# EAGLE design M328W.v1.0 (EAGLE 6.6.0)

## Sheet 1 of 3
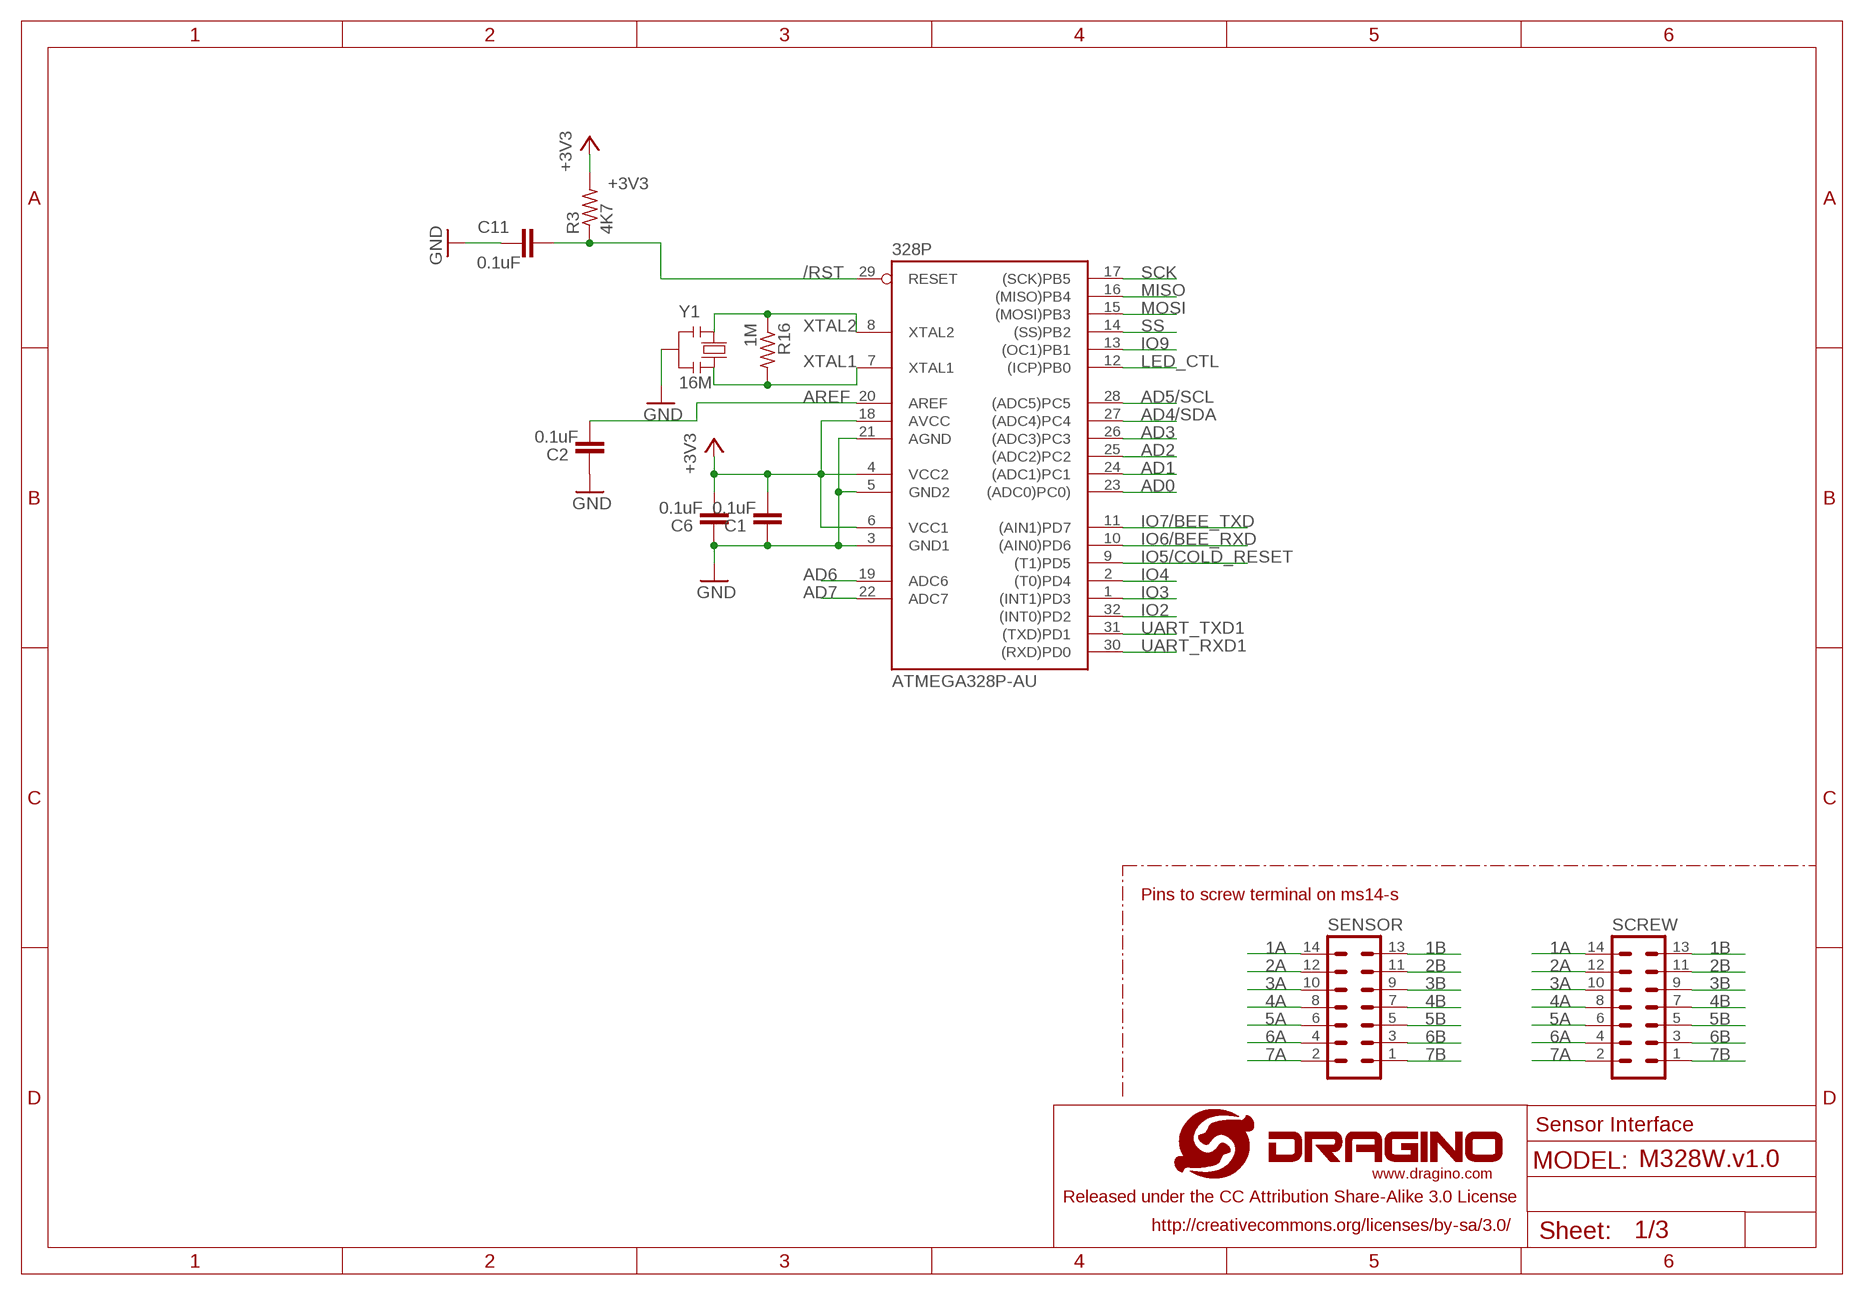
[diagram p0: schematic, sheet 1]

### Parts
328P  ATMEGA328P-AU  [TQFP32-08]
C1  0.1uF  C-EUC0402  [C0402]
C2  0.1uF  C-EUC0402  [C0402]
C6  0.1uF  C-EUC0402  [C0402]
C11  0.1uF  C-EUC0402  [C0402]
R3  4K7  R-US_R0402  [R0402]
R16  1M  R-US_R0402  [R0402]
SCREW  MA07-2  [MA07-2]
SENSOR  MA07-2  [MA07-2]
Y1  16M  RESONATORMU  [RESONATOR]

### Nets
1A: SCREW.14 SENSOR.14
1B: SCREW.13 SENSOR.13
2A: SCREW.12 SENSOR.12
2B: SCREW.11 SENSOR.11
3A: SCREW.10 SENSOR.10
3B: SCREW.9 SENSOR.9
4A: SCREW.8 SENSOR.8
4B: SCREW.7 SENSOR.7
5A: SCREW.6 SENSOR.6
5B: SCREW.5 SENSOR.5
6A: SCREW.4 SENSOR.4
6B: SCREW.3 SENSOR.3
7A: SCREW.2 SENSOR.2
7B: SCREW.1 SENSOR.1
+3V3: 328P.4(VCC2) 328P.6(VCC1) 328P.18(AVCC) C1.2 C6.2 R3.2 ; also sheet 2,3
/RST: 328P.29(RESET) C11.1 R3.1 ; also sheet 2
AD0: 328P.23((ADC0)PC0)) ; also sheet 2
AD1: 328P.24((ADC1)PC1) ; also sheet 2
AD2: 328P.25((ADC2)PC2) ; also sheet 2
AD3: 328P.26((ADC3)PC3) ; also sheet 2
AD4/SDA: 328P.27((ADC4)PC4) ; also sheet 2
AD5/SCL: 328P.28((ADC5)PC5) ; also sheet 2
AD6: 328P.19(ADC6)
AD7: 328P.22(ADC7)
AREF: 328P.20(AREF) C2.2 ; also sheet 2
GND [gnd]: 328P.3(GND1) 328P.5(GND2) 328P.21(AGND) C1.1 C2.1 C6.1 C11.2 Y1.2 ; also sheet 2,3
IO2: 328P.32((INT0)PD2) ; also sheet 2,3
IO3: 328P.1((INT1)PD3) ; also sheet 2
IO4: 328P.2((T0)PD4) ; also sheet 2
IO5/COLD_RESET: 328P.9((T1)PD5) ; also sheet 2
IO6/BEE_RXD: 328P.10((AIN0)PD6) ; also sheet 2,3
IO7/BEE_TXD: 328P.11((AIN1)PD7) ; also sheet 2,3
IO9: 328P.13((OC1)PB1) ; also sheet 2
LED_CTL: 328P.12((ICP)PB0) ; also sheet 2
MISO: 328P.16((MISO)PB4) ; also sheet 2,3
MOSI: 328P.15((MOSI)PB3) ; also sheet 2,3
SCK: 328P.17((SCK)PB5) ; also sheet 2,3
SS: 328P.14((SS)PB2) ; also sheet 2,3
UART_RXD1: 328P.30((RXD)PD0) ; also sheet 2
UART_TXD1: 328P.31((TXD)PD1) ; also sheet 2
XTAL1: 328P.7(XTAL1) R16.2 Y1.3
XTAL2: 328P.8(XTAL2) R16.1 Y1.1

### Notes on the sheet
- Pins to screw terminal on ms14-s
- Sensor Interface

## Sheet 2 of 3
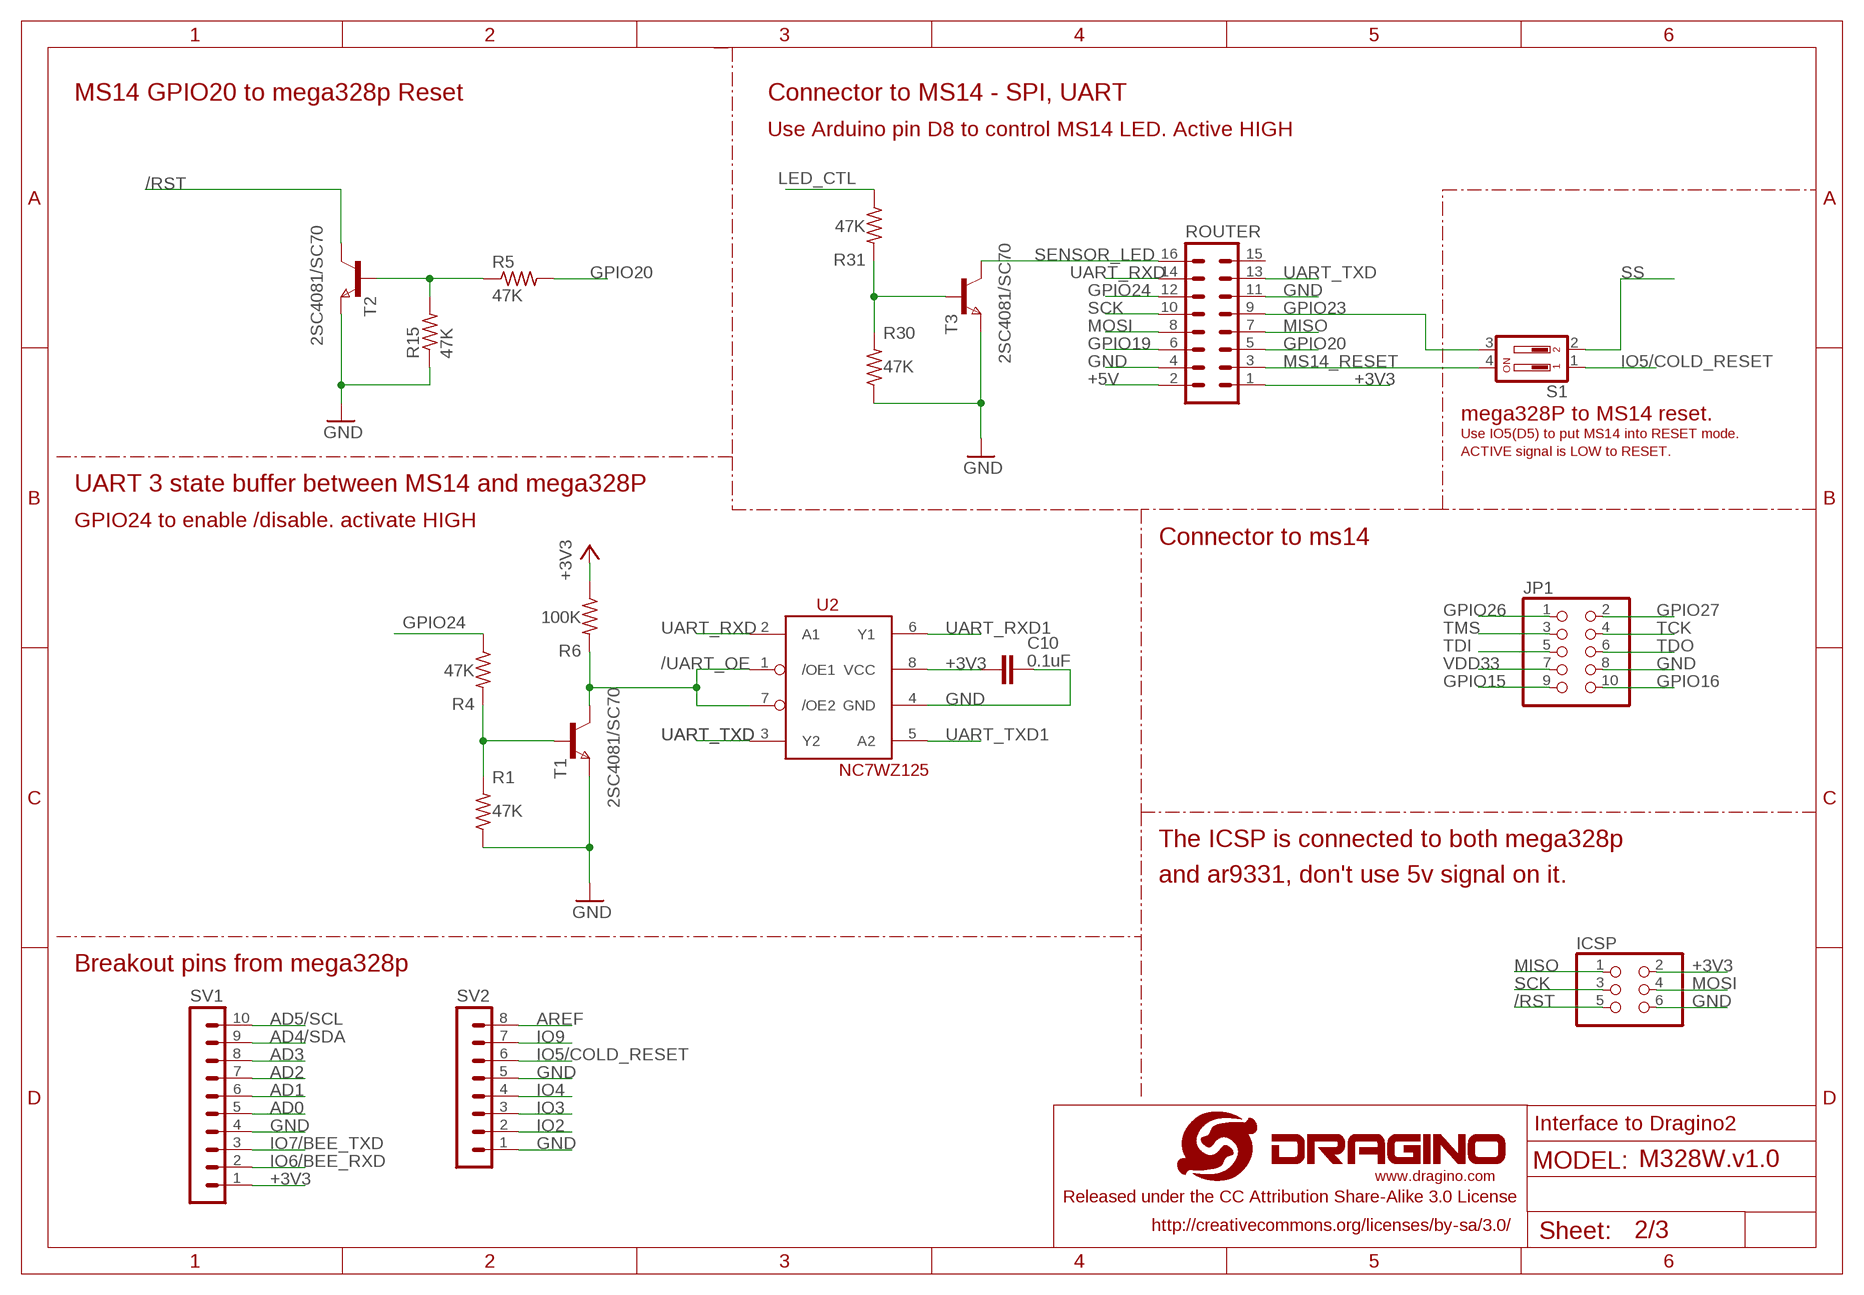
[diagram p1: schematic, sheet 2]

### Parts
C10  0.1uF  C-EUC0402  [C0402]
ICSP  PINHD-2X3  [2X03]
JP1  PINHD-2X5_2.00  [2X05M]
R1  47K  R-US_R0402  [R0402]
R4  47K  R-US_R0402  [R0402]
R5  47K  R-US_R0402  [R0402]
R6  100K  R-US_R0402  [R0402]
R15  47K  R-US_R0402  [R0402]
R30  47K  R-US_R0402  [R0402]
R31  47K  R-US_R0402  [R0402]
ROUTER  MA08-2  [MA08-2]
S1  DIP02YL  [DIP02YL]
SV1  MA10-1  [MA10-1]
SV2  MA08-1  [MA08-1]
T1  2SC4081/SC70  NPNSOT323  [SOT323]
T2  2SC4081/SC70  NPNSOT323  [SOT323]
T3  2SC4081/SC70  NPNSOT323  [SOT323]
U2  NC7WZ125  [US8]
U$5  LOGO-NEW  [LOGO-SILK-NEW]

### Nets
+3V3: C10.2 ICSP.2 R6.1 ROUTER.1 SV1.1 U2.8(VCC) ; also sheet 1,3
+5V: ROUTER.2
/RST: ICSP.5 T2.1(C) ; also sheet 1
/UART_OE: R6.2 T1.1(C) U2.1(/OE1) U2.7(/OE2)
AD0: SV1.5 ; also sheet 1
AD1: SV1.6 ; also sheet 1
AD2: SV1.7 ; also sheet 1
AD3: SV1.8 ; also sheet 1
AD4/SDA: SV1.9 ; also sheet 1
AD5/SCL: SV1.10 ; also sheet 1
AREF: SV2.8 ; also sheet 1
GND [gnd]: C10.1 ICSP.6 JP1.8 R1.1 R15.1 R30.1 ROUTER.4 ROUTER.11 SV1.4 SV2.1 SV2.5 T1.3(E) T2.3(E) T3.3(E) U2.4(GND) ; also sheet 1,3
GPIO15: JP1.9
GPIO16: JP1.10
GPIO19: ROUTER.6
GPIO20: R5.2 ROUTER.5
GPIO23: ROUTER.9 S1.3
GPIO24: R4.1 ROUTER.12
GPIO26: JP1.1 ; also sheet 3
GPIO27: JP1.2 ; also sheet 3
IO2: SV2.2 ; also sheet 1,3
IO3: SV2.3 ; also sheet 1
IO4: SV2.4 ; also sheet 1
IO5/COLD_RESET: S1.1 SV2.6 ; also sheet 1
IO6/BEE_RXD: SV1.2 ; also sheet 1,3
IO7/BEE_TXD: SV1.3 ; also sheet 1,3
IO9: SV2.7 ; also sheet 1
LED_CTL: R31.1 ; also sheet 1
MISO: ICSP.1 ROUTER.7 ; also sheet 1,3
MOSI: ICSP.4 ROUTER.8 ; also sheet 1,3
MS14_RESET: ROUTER.3 S1.4
N$4: R1.2 R4.2 T1.2(B)
N$8: R5.1 R15.2 T2.2(B)
N$9: R30.2 R31.2 T3.2(B)
SCK: ICSP.3 ROUTER.10 ; also sheet 1,3
SENSOR_LED: ROUTER.16 T3.1(C)
SS: S1.2 ; also sheet 1,3
TCK: JP1.4
TDI: JP1.5
TDO: JP1.6
TMS: JP1.3
UART_RXD: ROUTER.14 U2.2(A1) ; also sheet 3
UART_RXD1: U2.6(Y1) ; also sheet 1
UART_TXD: ROUTER.13 U2.3(Y2) ; also sheet 3
UART_TXD1: U2.5(A2) ; also sheet 1
VDD33: JP1.7
Unconnected: ROUTER.15

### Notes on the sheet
- MS14 GPIO20 to mega328p Reset | Connector to MS14 - SPI, UART
- Use Arduino pin D8 to control MS14 LED. Active HIGH
- mega328P to MS14 reset.
- Use IO5(D5) to put MS14 into RESET mode.
- ACTIVE signal is LOW to RESET.
- UART 3 state buffer between MS14 and mega328P
- GPIO24 to enable /disable. activate HIGH
- Connector to ms14
- The ICSP is connected to both mega328p
- and ar9331, don't use 5v signal on it.
- Breakout pins from mega328p
- Interface to Dragino2

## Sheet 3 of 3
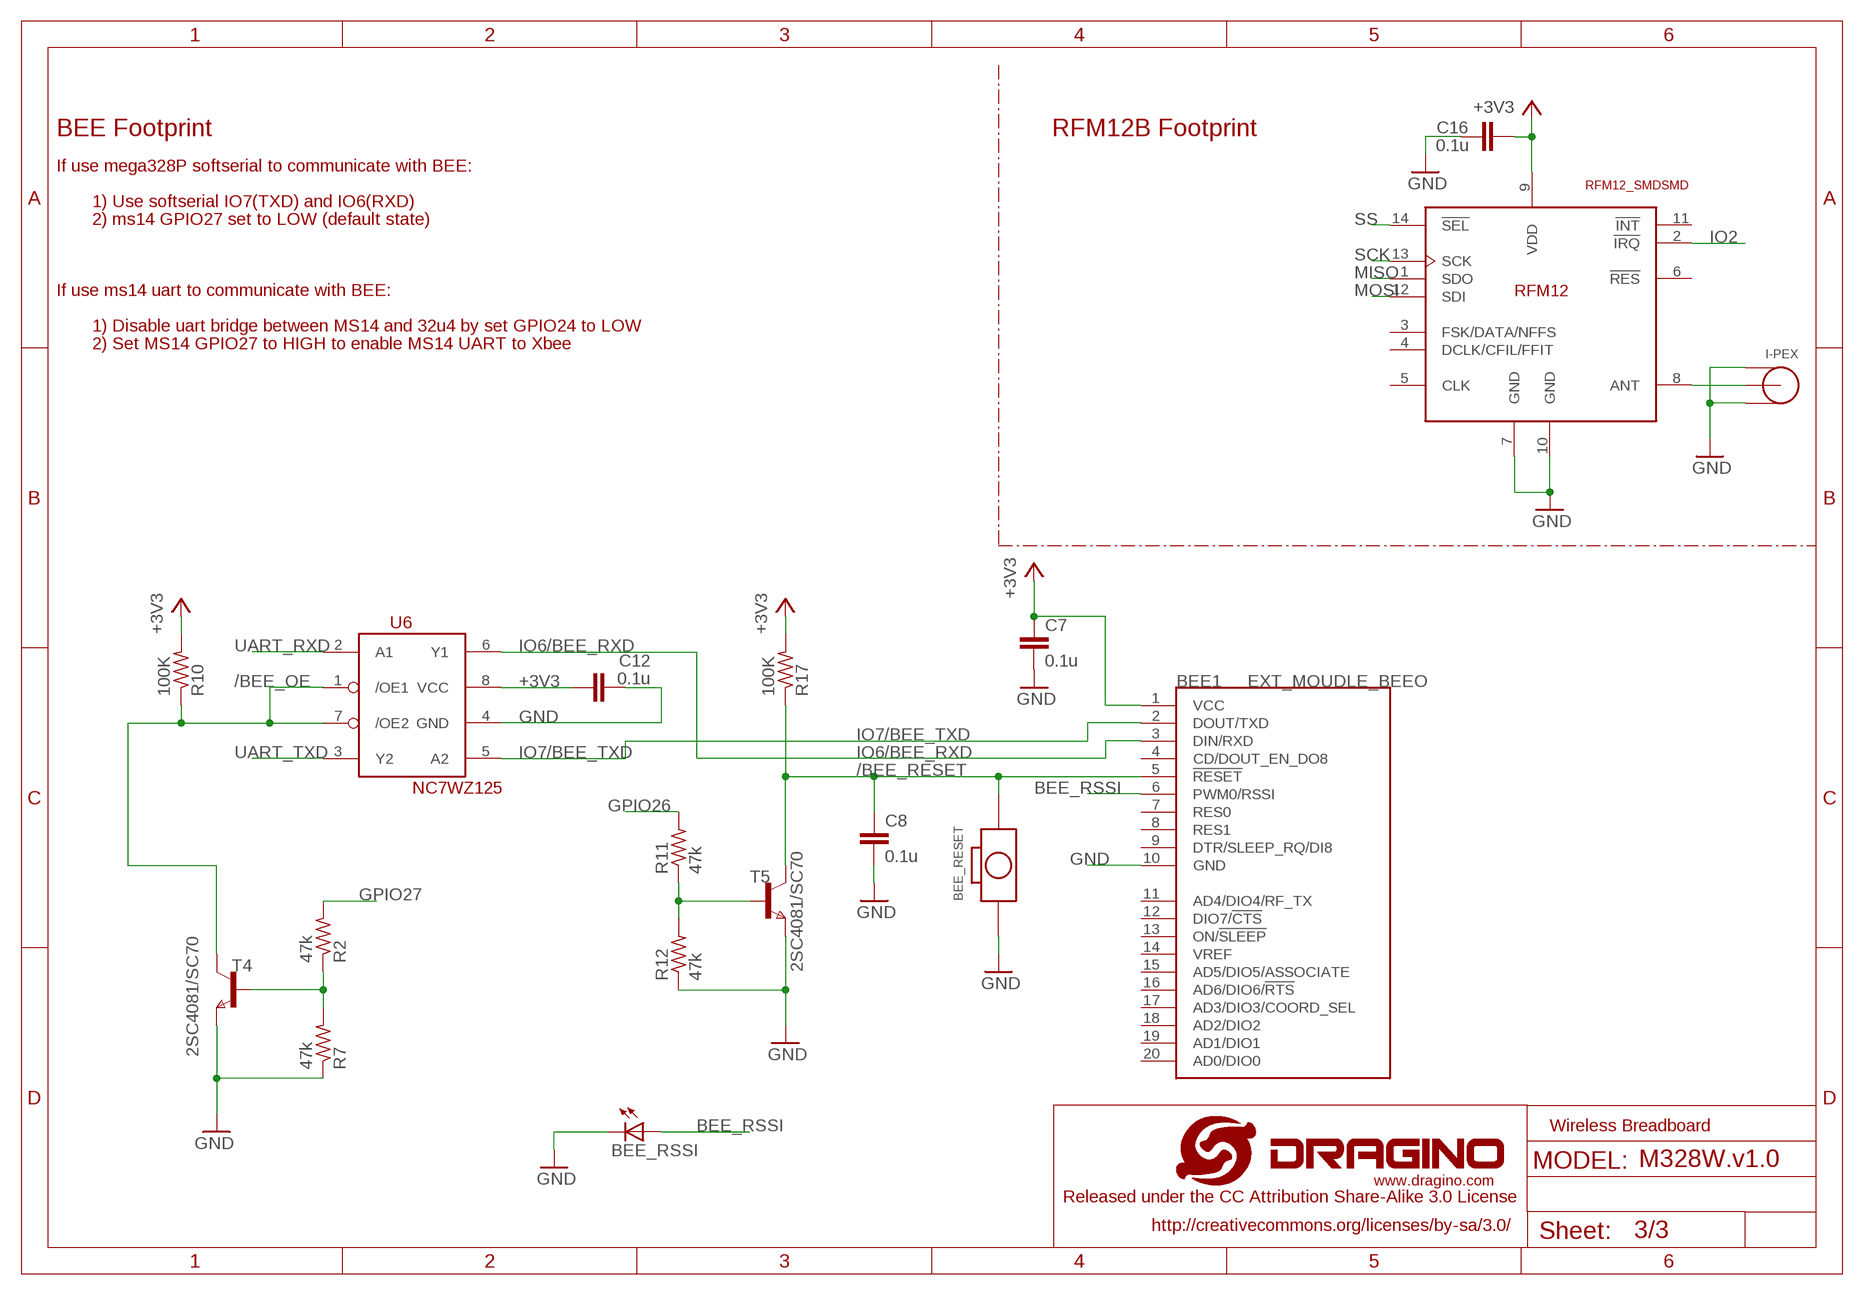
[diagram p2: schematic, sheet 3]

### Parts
BEE1  EXT_MOUDLE_BEEO  [EXT_MOUDLE_BEE]
BEE_RESET  CPT_SMD_BOTTON_1_SMD  [CPT_SMD_BOTTON_1]
BEE_RSSI  LEDCHIP-LED0805  [CHIP-LED0805]
C7  0.1u  C-EUC0402  [C0402]
C8  0.1u  C-EUC0402  [C0402]
C12  0.1u  C-EUC0402  [C0402]
C16  0.1u  C-EUC0402  [C0402]
I-PEX  I-PEX  [I-PEX]
R2  47k  R-US_R0402  [R0402]
R7  47k  R-US_R0402  [R0402]
R10  100K  R-US_R0402  [R0402]
R11  47k  R-US_R0402  [R0402]
R12  47k  R-US_R0402  [R0402]
R17  100K  R-US_R0402  [R0402]
T4  2SC4081/SC70  NPNSOT323  [SOT323]
T5  2SC4081/SC70  NPNSOT323  [SOT323]
U6  NC7WZ125  [US8]
U$3  RFM12_SMDSMD  [RFM12]

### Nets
+3V3: BEE1.1(VCC) C7.1 C12.1 C16.2 R10.2 R17.2 U6.8(VCC) U$3.9(VDD) ; also sheet 1,2
/BEE_OE: R10.1 T4.1(C) U6.1(/OE1) U6.7(/OE2)
/BEE_RESET: BEE1.5(!RESET) BEE_RESET.P$2 C8.1 R17.1 T5.1(C)
BEE_RSSI: BEE1.6(PWM0/RSSI) BEE_RSSI.A
GND [gnd]: BEE1.10(GND) BEE_RESET.1 BEE_RSSI.C C7.2 C8.2 C12.2 C16.1 I-PEX.GND I-PEX.GND1 R7.1 R12.1 T4.3(E) T5.3(E) U6.4(GND) U$3.7(GND) U$3.10(GND) ; also sheet 1,2
GPIO26: R11.2 ; also sheet 2
GPIO27: R2.2 ; also sheet 2
IO2: U$3.2(!IRQ) ; also sheet 1,2
IO6/BEE_RXD: BEE1.3(DIN/RXD) U6.6(Y1) ; also sheet 1,2
IO7/BEE_TXD: BEE1.2(DOUT/TXD) U6.5(A2) ; also sheet 1,2
MISO: U$3.1(SDO) ; also sheet 1,2
MOSI: U$3.12(SDI) ; also sheet 1,2
N$11: R2.1 R7.2 T4.2(B)
N$12: R11.1 R12.2 T5.2(B)
N$16: I-PEX.SIG U$3.8(ANT)
SCK: U$3.13(SCK) ; also sheet 1,2
SS: U$3.14(!SEL) ; also sheet 1,2
UART_RXD: U6.2(A1) ; also sheet 2
UART_TXD: U6.3(Y2) ; also sheet 2
Unconnected: BEE1.4(CD/DOUT_EN_DO8) BEE1.7(RES0) BEE1.8(RES1) BEE1.9(DTR/SLEEP_RQ/DI8) BEE1.11(AD4/DIO4/RF_TX) BEE1.12(DIO7/!CTS) BEE1.13(ON/!SLEEP) BEE1.14(VREF) BEE1.15(AD5/DIO5/ASSOCIATE) BEE1.16(AD6/DIO6/!RTS) BEE1.17(AD3/DIO3/COORD_SEL) BEE1.18(AD2/DIO2) BEE1.19(AD1/DIO1) BEE1.20(AD0/DIO0) U$3.3(FSK/DATA/NFFS) U$3.4(DCLK/CFIL/FFIT) U$3.5(CLK) U$3.6(!RES) U$3.11(!INT)

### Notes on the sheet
- BEE Footprint | RFM12B Footprint
- If use mega328P softserial to communicate with BEE:
- 1) Use softserial IO7(TXD) and IO6(RXD)
- 2) ms14 GPIO27 set to LOW (default state)
- If use ms14 uart to communicate with BEE:
- 1) Disable uart bridge between MS14 and 32u4 by set GPIO24 to LOW
- 2) Set MS14 GPIO27 to HIGH to enable MS14 UART to Xbee
- Wireless Breadboard

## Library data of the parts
328P = dragino:ATMEGA328P-: MICROCONTROLLER 4 Kbytes FLASH 128 bytes SRAM 256 bytes EEPROM UART 6-channel 10 bit ADC
BEE1 = Bees_Shield:EXT_MOUDLE_BEE
BEE_RESET = Bees_Shield:CPT_SMD_BOTTON_1
BEE_RSSI = dragino:LED: LED
C1 C2 C6-C8 C10-C12 C16 = dragino:C-EU: CAPACITOR, European symbol
I-PEX = dragino:I-PEX: I-PEX connector
ICSP = dragino:PINHD-2X3: PIN HEADER
JP1 = dragino:PINHD-2X5: PIN HEADER
R1-R7 R10-R12 R15-R17 R30 R31 = dragino:R-US_: RESISTOR, American symbol
ROUTER = dragino:MA08-2: PIN HEADER; OC_FARNELL: unknown; OC_NEWARK: unknown
S1 = switch-dil:DIP02YL: DIL/CODE SWITCH; OC_FARNELL: unknown; OC_NEWARK: unknown
SCREW SENSOR = dragino:MA07-2: PIN HEADER; OC_FARNELL: unknown; OC_NEWARK: unknown
SV1 = con-lstb:MA10-1: PIN HEADER; OC_FARNELL: unknown; OC_NEWARK: unknown
SV2 = con-lstb:MA08-1: PIN HEADER; OC_FARNELL: unknown; OC_NEWARK: unknown
T1-T5 = zetex:NPNSOT323: NPN TRANSISTOR; MPN: DSS4160U-7; OC_FARNELL: 1710696; OC_NEWARK: 25R4558
U2 U6 = dragino:NC7WZ125: 3 state buffer: http://www.fairchildsemi.com/ds/NC/NC7WZ125.pdf
U$3 = dragino:RFM12_SMD: RFM12 is a low costing ISM band transceiver module implemented with unique PLL. It works signal ranges from 315/433/868/915MHZ bands, comply with FCC, ETSI regulation. The SPI interface is used to communicate with microcontroller for parameter setting.
U$5 = dragino:LOGO-NEW
Y1 = SmartPrj:RESONATOR

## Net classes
0 default: width 0.203 mm, clearance 0.254 mm
1 power: width 0.61 mm, drill 0.61 mm, clearance 0.254 mm
2 gnd: width 0.305 mm, drill 0.33 mm, clearance 0.254 mm
3 usbvcc: width 0.508 mm, drill 0.61 mm, clearance 0.254 mm
4 aref: width 0.406 mm, drill 0.61 mm, clearance 0.254 mm
5 usbtrace: width 0.254 mm, clearance 0.152 mm

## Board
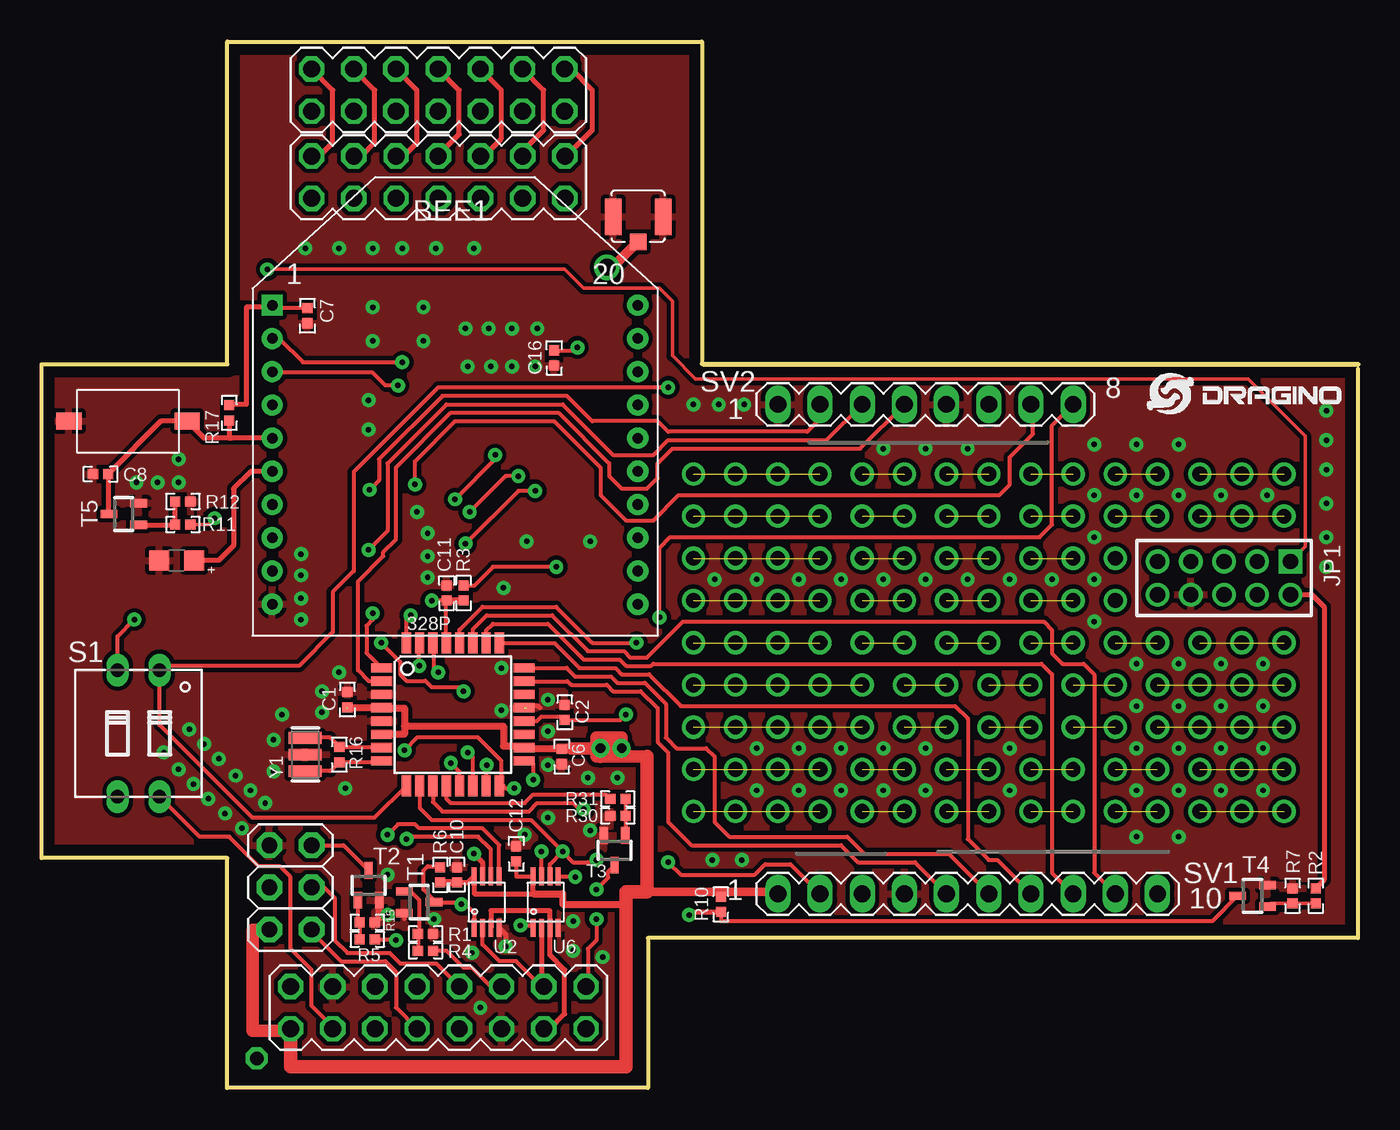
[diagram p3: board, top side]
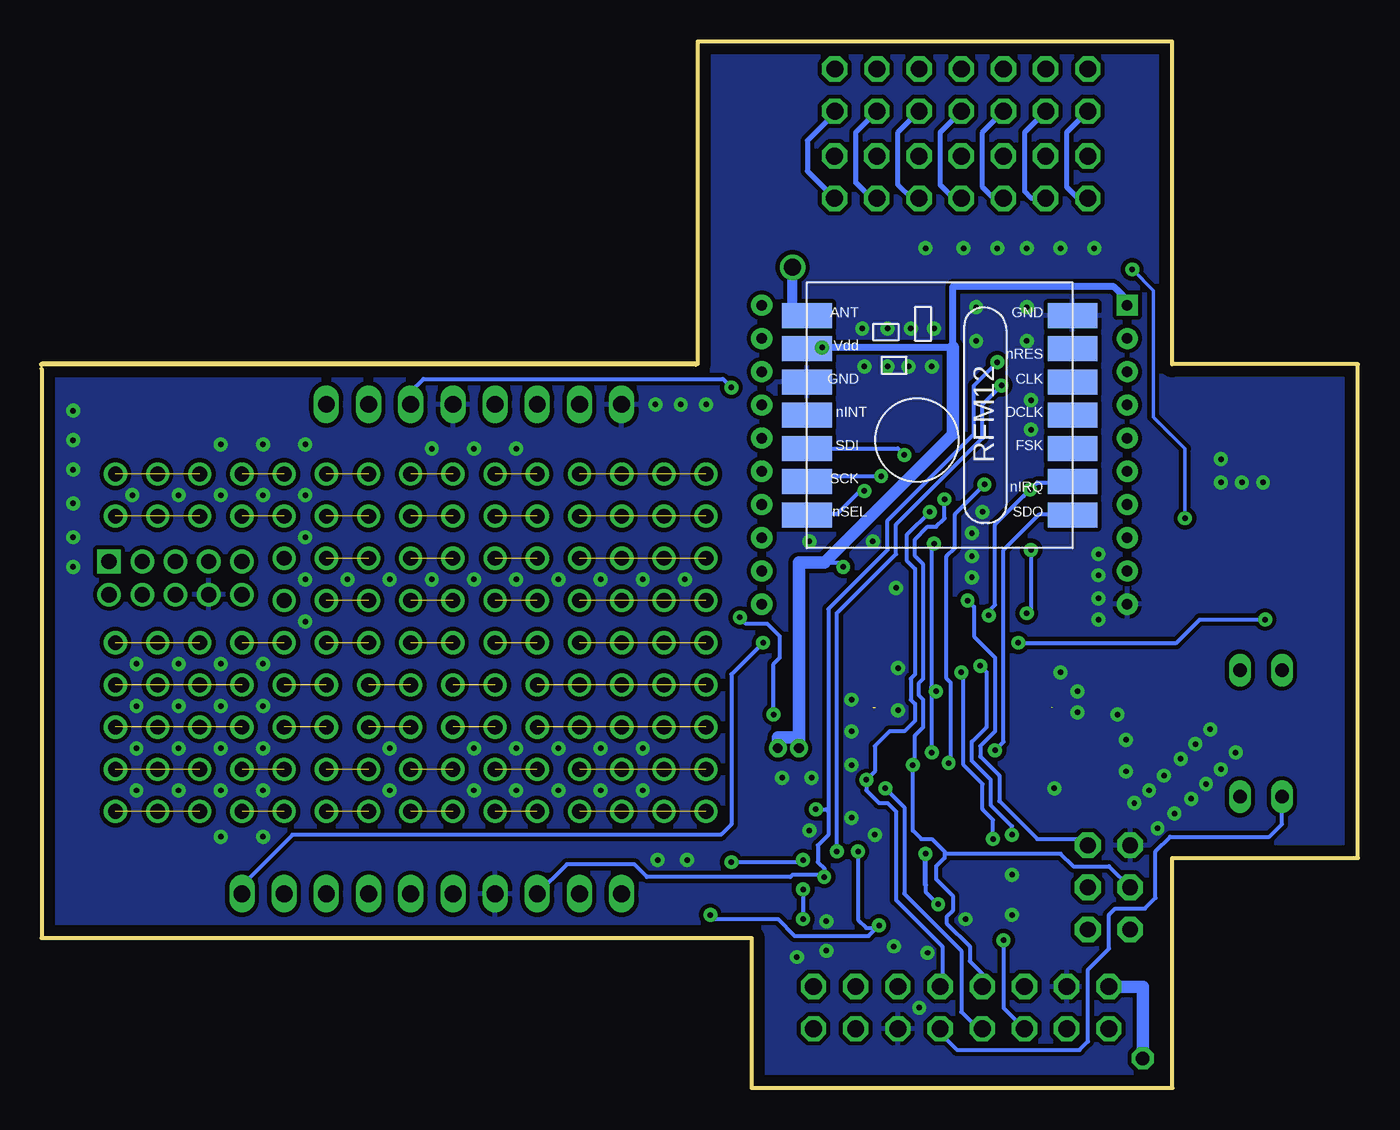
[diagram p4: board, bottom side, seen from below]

Size 79.25 x 63.01 mm. Coordinates in mm from the lower left corner, seen from the top.
Outline: 39.75,43.61 39.75,63.01 11.18,63.01 11.18,43.58 0,43.58 0,13.86 11.18,13.86 11.18,0
Outline: 79.25,43.3 79.25,9.03 36.51,9.03 36.51,0.02 11.16,0.02
Outline: 39.88,43.58 79.25,43.58
Copper layers (1*16): Top 0.035mm / dielectric 1.5mm / Bottom 0.035mm
Design rules "default *": minimum track width 5mil, minimum drill 10mil, track to track 6mil, track to pad 7mil, pad to pad 7mil, via to via 10mil, smd to smd 7mil, copper to edge 26mil, drill to drill 10mil, minimum pad ring 10mil, minimum via ring 10mil, stop-mask expansion 1mil, vias tented up to drill 30mil, thermal gap 10mil

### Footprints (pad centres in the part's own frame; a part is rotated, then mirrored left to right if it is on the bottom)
TQFP32-08 = smd 1.27 x 0.559: 1 -4.293,2.8; 2 -4.293,2; 3 -4.293,1.2; 4 -4.293,0.4; 5 -4.293,-0.4; 6 -4.293,-1.2; 7 -4.293,-2; 8 -4.293,-2.8; 17 4.293,-2.8; 18 4.293,-2; 19 4.293,-1.2; 20 4.293,-0.4; 21 4.293,0.4; 22 4.293,1.2; 23 4.293,2; 24 4.293,2.8 | smd 0.559 x 1.27: 9 -2.8,-4.293; 10 -2,-4.293; 11 -1.2,-4.293; 12 -0.4,-4.293; 13 0.4,-4.293; 14 1.2,-4.293; 15 2,-4.293; 16 2.8,-4.293; 25 2.8,4.293; 26 2,4.293; 27 1.2,4.293; 28 0.4,4.293; 29 -0.4,4.293; 30 -1.2,4.293; 31 -2,4.293; 32 -2.8,4.293
EXT_MOUDLE_BEE = drill 0.635 pad 1.27 square: 1 -11,0 | drill 0.635 pad 1.27: 2 -11,-2; 3 -11,-4; 4 -11,-6; 5 -11,-8; 6 -11,-10; 7 -11,-12; 8 -11,-14; 9 -11,-16; 10 -11,-18; 11 11,-18; 12 11,-16; 13 11,-14; 14 11,-12; 15 11,-10; 16 11,-8; 17 11,-6; 18 11,-4; 19 11,-2; 20 11,0
CPT_SMD_BOTTON_1 = smd 1.524 x 1.016: 1 -3.556,0; P$2 3.556,0
CHIP-LED0805 = smd 1.2 x 1.2: A 0,-1.05; C 0,1.05
C0402 = smd 0.61 x 0.61: 1 -0.457,0; 2 0.457,0
I-PEX = smd 1 x 2.2: GND -1.65,-0.27; GND1 1.35,-0.27 | smd 1 x 1: SIG -0.15,-1.77
2X03 = drill 0.95 pad 1.55 octagon: 1 -2.54,-1.27; 2 -2.54,1.27; 3 0,-1.27; 4 0,1.27; 5 2.54,-1.27; 6 2.54,1.27
2X05M = drill 0.914 square: 1 -4,-1 | drill 0.914: 2 -4,1; 3 -2,-1; 4 -2,1; 5 0,-1; 6 0,1; 7 2,-1; 8 2,1; 9 4,-1; 10 4,1
R0402 = smd 0.61 x 0.61: 1 -0.457,0; 2 0.457,0
MA08-2 = drill 1.016 octagon: 1 -8.89,-1.27; 2 -8.89,1.27; 3 -6.35,-1.27; 4 -6.35,1.27; 5 -3.81,-1.27; 6 -3.81,1.27; 7 -1.27,-1.27; 8 -1.27,1.27; 9 1.27,-1.27; 10 1.27,1.27; 11 3.81,-1.27; 12 3.81,1.27; 13 6.35,-1.27; 14 6.35,1.27; 15 8.89,-1.27; 16 8.89,1.27
DIP02YL = drill 0.813 long: 1 -1.27,-3.81; 2 1.27,-3.81; 3 1.27,3.81; 4 -1.27,3.81
MA07-2 = drill 1.016 octagon: 1 -7.62,-1.27; 2 -7.62,1.27; 3 -5.08,-1.27; 4 -5.08,1.27; 5 -2.54,-1.27; 6 -2.54,1.27; 7 0,-1.27; 8 0,1.27; 9 2.54,-1.27; 10 2.54,1.27; 11 5.08,-1.27; 12 5.08,1.27; 13 7.62,-1.27; 14 7.62,1.27
MA10-1 = drill 1.016 long: 1 -11.43,0; 2 -8.89,0; 3 -6.35,0; 4 -3.81,0; 5 -1.27,0; 6 1.27,0; 7 3.81,0; 8 6.35,0; 9 8.89,0; 10 11.43,0
MA08-1 = drill 1.016 long: 1 -8.89,0; 2 -6.35,0; 3 -3.81,0; 4 -1.27,0; 5 1.27,0; 6 3.81,0; 7 6.35,0; 8 8.89,0
SOT323 = smd 0.5 x 1: 1 0,0.9; 2 -0.65,-0.9; 3 0.65,-0.9
US8 = smd 0.3 x 1.1: 1 -0.75,-1.55; 2 -0.25,-1.55; 3 0.25,-1.55; 4 0.75,-1.55; 5 0.75,1.55; 6 0.25,1.55; 7 -0.25,1.55; 8 -0.75,1.55
RFM12 = smd 1.5 x 3: 1 -5,-10; 2 -3,-10; 3 -1,-10; 4 1,-10; 5 3,-10; 6 5,-10; 7 7,-10; 8 7,6; 9 5,6; 10 3,6; 11 1,6; 12 -1,6; 13 -3,6; 14 -5,6
RESONATOR = smd 0.7 x 2: 1 -1,0; 2 0,0; 3 1,0

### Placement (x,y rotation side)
328P  24.77,22.5 0 top
BEE1  24.89,47.13 0 top
BEE_RESET  5.21,40.15 0 top
BEE_RSSI  8.13,31.77 90 top
C1  18.41,23.38 270 top
C2  31.5,22.62 270 top
C6  31.32,19.96 90 top
C7  16,46.5 270 top
C8  3.56,36.97 180 top
C10  25.02,12.84 270 top
C11  24.38,29.81 90 top
C12  28.57,14.11 90 top
C16  30.86,43.96 90 top
I-PEX  36.07,52.72 0 top
ICSP  14.99,12.08 90 top
JP1  71.18,30.71 180 top
R1  23.11,9.29 180 top
R2  76.71,11.57 90 top
R3  25.4,29.81 90 top
R4  23.11,8.27 180 top
R5  19.61,8.96 0 top
R6  24,12.84 90 top
R7  75.31,11.57 270 top
R10  40.89,11.07 90 top
R11  8.51,33.93 0 top
R12  8.51,35.32 180 top
R15  19.61,9.97 180 top
R16  17.93,20.07 90 top
R17  11.3,40.66 90 top
R30  34.7,16.39 0 top
R31  34.7,17.41 0 top
ROUTER  23.88,4.84 0 top
S1  5.84,21.35 180 top
SCREW  23.88,60.09 0 top
SENSOR  23.88,54.84 0 top
SV1  55.75,11.7 0 top
SV2  53.21,41.16 0 top
T1  22.73,11.19 270 top
T2  19.68,12.21 0 top
T3  34.5,14.31 180 top
T4  72.9,11.57 90 top
T5  4.95,34.56 90 top
U2  26.8,11.19 0 top
U6  30.35,11.19 0 top
U$3  27.18,39.51 90 bottom
U$5  66.53,40.58 0 top
Y1  15.88,20.08 90 top

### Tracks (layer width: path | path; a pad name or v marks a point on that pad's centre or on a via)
1A
  Top 0.305: SCREW.14 31.88,61.36 33.15,60.09 33.15,57.67 31.5,56.02 31.5,56.1 SENSOR.14
1B
  Bottom 0.305: SCREW.13 31.5,58.69 33.15,57.04 33.15,55.22 SENSOR.13
2A
  Top 0.305: SENSOR.12 28.96,56.41 30.23,57.67 30.23,60.09 SCREW.12
2B
  Bottom 0.305: SENSOR.11 29.3,53.57 30.23,54.5 30.23,57.55 SCREW.11
3A
  Top 0.305: SENSOR.10 26.63,56.11 27.69,57.17 27.69,60.09 SCREW.10
3B
  Bottom 0.305: SENSOR.9 26.89,53.57 27.69,54.37 27.69,57.55 SCREW.9
4A
  Top 0.305: SENSOR.8 23.88,56.16 25.15,57.42 25.15,60.09 SCREW.8
4B
  Bottom 0.305: SENSOR.7 24.35,53.57 25.15,54.37 25.15,57.55 SCREW.7
5A
  Top 0.305: SENSOR.6 21.81,56.11 22.61,56.91 22.61,60.09 SCREW.6
5B
  Bottom 0.305: SENSOR.5 21.93,53.57 22.61,54.25 22.61,57.55 SCREW.5
6A
  Top 0.305: SENSOR.4 19.27,56.11 20.07,56.91 20.07,60.09 SCREW.4
6B
  Bottom 0.305: SENSOR.3 19.65,53.57 20.07,53.99 20.07,57.55 SCREW.3
7A
  Top 0.305: SENSOR.2 16.73,56.11 17.53,56.91 17.53,60.09 SCREW.2
7B
  Bottom 0.305: SENSOR.1 16.85,53.57 17.53,54.25 17.53,57.55 SCREW.1
+3V3  (via drill 0.33, 0.58)  (1 unrouted)
  Top 0.254: C12.1 28.57,12.74 U6.8 | C7.1 14.07,46.96 BEE1.1 | C16.2 32.08,44.42 v32.26,44.59 | v30.99,31.39 27.18,31.39 26.04,30.24 25.43,30.24 R3.2 | R10.2 40.89,11.83
  Top 0.305: BEE1.1 13.89,47.01 12.32,47.01 12.32,41.16 11.3,41.16 R17.2 | C10.2 25.69,12.39 U2.8 26.05,11.7 29.59,11.7 U6.8
  Top 0.406: 21.84,21.8 21.84,22.88 20.47,22.88 328P.4 18.41,22.9 | 20.57,21.23 20.47,21.23 328P.6 21.84,21.3 21.84,21.8 | R6.1 C10.2 | 29.59,11.7 31.37,11.7 31.37,11.07 35.18,11.07 35.18,11.57 | 21.84,21.8 27.81,21.8 27.81,20.59 29.06,20.59 328P.18 29.13,20.42 C6.2 31.36,20.46 31.88,20.46
  Top 0.508: 36.45,11.83 40.89,11.83 44.2,11.83 SV1.1 | 33.66,20.21 v33.66,20.46 33.66,20.5
  Top 0.762: ICSP.2 12.7,9.54 12.7,3.45 14.99,3.45 ROUTER.1 | 33.66,19.96 34.93,19.96 34.93,21.1 33.4,21.1 33.4,20.46 | 33.4,19.96 33.4,20.46 | 33.4,20.46 v33.66,20.46 34.42,20.46 34.42,19.96 36.45,19.96 | 33.4,20.46 31.88,20.46
  Top 0.813: ROUTER.1 14.99,1.29 35.18,1.29 35.18,11.57 35.18,11.83 36.45,11.83 36.45,19.96 | 33.66,19.96 33.66,20.21
  Bottom 0.254: 32.13,31.64 31.24,31.64 v30.99,31.39
  Bottom 0.406: U$3.9 33.1,44.59 v32.26,44.59 24.38,44.59 24.38,48.28 14.73,48.28 13.89,47.44 BEE1.1
  Bottom 0.762: v33.66,20.46 33.66,21.1 | 33.66,21.1 33.66,31.64 32.13,31.64 24.38,39.39 24.38,44.59 | v34.93,20.46 34.93,21.1 33.66,21.1
+5V  (via drill 0.81)
  Bottom 0.762: ROUTER.2 12.95,6.11 v12.95,1.79
/BEE_OE  (via drill 0.33)
  Top 0.254: T4.1 70.48,10.05 40.89,10.05 R10.1 | U6.7 v30.1,14.24 | v28.83,9.8 29.45,9.8 U6.1
  Top 0.305: v38.99,10.43 39.17,10.61 R10.1
  Bottom 0.254: v38.99,10.43 38.73,10.18 34.93,10.18 33.91,9.16 29.46,9.16 28.98,9.64 | v30.1,14.24 30.1,10.14 U6.1 28.98,9.64 | 28.98,9.64 v28.83,9.8
/BEE_RESET
  Top 0.305: BEE1.5 11.43,39.13 11.3,39.13 | 11.3,39.13 9.78,39.13 BEE_RESET.P$2 7.19,40.15 C8.1 4.01,34.6 T5.1 | R17.1 11.3,39.13
/RST  (via drill 0.33)
  Top 0.254: ICSP.5 18.17,14.62 T2.1 | 328P.29 24.36,29.33 C11.1 v23.49,29.35
  Top 0.406: C11.1 R3.1
  Bottom 0.254: v23.49,29.35 23.11,28.97 23.11,27.19 21.84,25.92 21.84,21.48 22.73,20.59 22.73,19.96 21.59,18.81 21.59,17.29 19.3,15 16.64,15 ICSP.5
/UART_OE  (via drill 0.33)
  Top 0.254: U2.7 | R6.2 23.95,13.35 23.24,13.35 22.99,13.1 22.99,11.95 23.63,11.31 T1.1 25.15,11.19 v25.27,11.07 25.53,11.07 26.04,10.56 26.04,9.65 U2.1
  Top 0.305: v26.04,14.11 26.55,13.6 U2.7
  Bottom 0.254: 26.04,12.21 26.04,11.83 v25.27,11.07
  Bottom 0.305: 26.04,12.21 v26.04,14.11
AD0
  Top 0.254: 328P.23 31.65,24.5 31.88,24.27 34.04,24.27 34.42,23.89 36.07,23.89 37.08,22.88 37.08,20.84 37.72,20.21 37.72,16.02 39.12,14.62 48.13,14.62 49.15,13.61 52.58,13.61 SV1.5
AD1
  Top 0.254: 328P.24 31.62,25.3 32.13,24.78 34.29,24.78 34.67,24.4 36.32,24.4 37.59,23.13 37.59,21.1 38.23,20.46 40.01,20.46 40.51,19.96 40.51,16.02 41.4,15.13 48.51,15.13 49.53,14.11 54.61,14.11 SV1.6
AD2
  Top 0.254: 328P.25 30.89,26.79 32.38,25.29 34.54,25.29 34.93,24.91 36.58,24.91 38.48,23 54.99,23 55.75,22.24 55.75,15 57.02,13.73 57.53,13.73 SV1.7
AD3
  Top 0.254: 328P.26 26.77,27.54 27.18,27.96 30.48,27.96 32.64,25.8 34.8,25.8 35.18,25.42 36.7,25.42 36.83,25.54 60.2,25.54 60.83,24.91 60.83,12.97 SV1.8
AD4/SDA
  Top 0.254: 328P.27 25.96,27.63 26.8,28.46 30.73,28.46 32.89,26.31 35.05,26.31 35.43,25.92 36.45,25.92 38.61,28.08 60.33,28.08 60.83,27.58 60.83,26.18 61.47,25.54 62.74,25.54 63.37,24.91 63.37,12.97 SV1.9
AD5/SCL  (via drill 0.33)
  Top 0.254: 328P.28 25.16,27.59 26.54,28.97 30.99,28.97 33.15,26.81 v35.81,26.81
  Bottom 0.254: v35.81,26.81 37.72,24.91 37.72,15.89 38.35,15.26 64.14,15.26 67.18,12.21 SV1.10
AREF  (via drill 0.33)
  Top 0.254: 328P.20 29.83,22.1 30.1,22.37 31.29,22.37 C2.2 34.85,22.17 v35.18,22.5 | v37.21,28.34 37.21,32.53 37.85,33.16 60.07,33.16 60.83,33.93 60.83,39.89 SV2.8
  Bottom 0.254: v35.18,22.5 35.18,25.54 34.8,25.92 34.8,27.19 35.56,27.96 36.83,27.96 v37.21,28.34
BEE_RSSI
  Top 0.305: BEE1.6 12.61,37.13 11.56,36.08 11.56,32.66 10.67,31.77 BEE_RSSI.A
GND  (via drill 0.33)  (1 unrouted)
  Top 0.254: T1.3 21.83,10.19 21.84,10.18 21.84,10.56 | R1.1 23.62,9.29
  Top 0.305: U2.4 27.94,9.25 v27.94,8.53 | 29.99,22.9 29.88,23 29.59,23 29.46,22.88 29.21,22.88
  Top 0.406: R15.1 20.34,10.24 T2.3
  other vias: 20.83,10.43 32,8.27 25.91,8.14 33.78,7.89 32,10.05 29.08,15.26 33.02,15.51 30.48,16.27 30.48,19.45 30.48,23.38 30.48,21.48 32.89,18.69 34.67,18.69 11.68,18.81 10.67,19.83 12.57,17.92 13.46,17.16 9.78,20.72 8.89,21.61 7.37,20.21 8.25,19.19 9.14,18.3 10.03,17.42 11.05,16.53 12.07,15.64 5.71,36.47 6.99,36.47 8.25,36.47 8.25,37.86 39.24,41.16 40.77,41.16 42.29,41.16 29.72,43.45 28.32,43.45 27.05,43.45 25.65,43.45 29.84,45.74 28.32,45.74 26.92,45.74 25.53,45.74 13.97,20.97 13.97,19.07 14.48,22.5 16.89,22.62 18.29,18.05 23.24,30.75 23.24,32.02 23.24,33.42 22.61,34.69 15.62,28.21 15.62,29.48 15.62,30.88 15.62,32.15 17.91,25.04 16.89,23.89 40.39,13.73 42.16,13.73 43.05,17.92 45.59,17.92 48.13,17.92 50.67,17.92 53.21,17.92 58.29,17.92 58.29,20.46 53.21,20.46 50.67,20.46 48.13,20.46 45.59,20.46 43.05,20.46 65.91,17.92 68.45,17.92 70.99,17.92 65.91,20.46 68.45,20.46 70.99,20.46 73.53,20.46 73.53,17.92 73.53,23 70.99,23 68.45,23 65.91,23 65.91,25.54 68.45,25.54 70.99,25.54 73.53,25.54 63.37,28.08 63.37,30.62 63.37,33.16 60.83,30.62 58.29,30.62 55.75,30.62 53.21,30.62 50.67,30.62 48.13,30.62 45.59,30.62 43.05,30.62 40.51,30.62 63.37,35.7 65.91,35.7 68.45,35.7 70.99,35.7 73.79,35.7 77.34,40.78 77.34,39.01 77.34,37.23 77.34,35.2 77.34,33.16 77.34,31.39 65.91,15.13 68.45,15.13 50.67,38.5 53.21,38.5 55.75,38.5 63.37,38.75 65.91,38.75 68.45,38.75 22.99,47.01 19.94,47.01 19.94,44.97 22.99,44.97 15.88,50.56 17.91,50.56 19.94,50.56 21.72,50.56 23.75,50.56 26.04,50.56 19.68,41.42 19.68,39.64 29.21,32.91 33.02,32.91 27.69,22.75 27.69,25.29 27.81,30.12 20.83,12.84 26.42,4.84 23.62,10.18
  pour Top (rank 2): 11.18,43.58 11.18,63.04 39.75,62.91 39.75,43.58 79.02,43.58 79.27,9.03 43.69,8.94 36.56,8.89 36.7,0.4 12.07,0.27 11.05,0.27 11.05,13.86 0,13.86 0,13.99 0.13,43.58
  pour Bottom (rank 2): 0.13,43.45 0,13.86 11.18,13.86 11.18,0.4 11.3,0.4 36.58,0.27 36.44,8.93 79.27,9.03 79.02,43.62 39.7,43.62 39.75,63.01 10.92,63.01 11.43,43.32
GPIO20  (via drill 0.33)
  Top 0.254: R5.2 21.29,8.96 v21.34,8.91
  Bottom 0.254: v21.34,8.91 21.34,4.83 ROUTER.5
GPIO23
  Bottom 0.254: ROUTER.9 25.15,3.33 24.13,2.3 16.76,2.3 16.26,2.81 16.26,7.13 14.99,8.4 14.99,10.43 14.61,10.81 12.83,10.81 12.19,11.45 12.19,14.24 11.3,15.13 5.33,15.13 4.57,15.89 S1.3
GPIO24
  Top 0.254: ROUTER.12 27.05,6.11 25.91,7.26 25.4,7.26 24.38,8.27 R4.1
GPIO26  (via drill 0.33)
  Top 0.203: R11.2 10.03,33.93 v10.41,34.31 | v13.59,49.29 31.5,49.29 32.64,48.15 37.21,48.15 37.97,47.39 37.97,44.09 39.37,42.69 72.64,42.69 76.07,39.26 76.07,32.6 JP1.1
  Bottom 0.203: v10.41,34.31 10.41,38.5 12.32,40.4 12.32,48.02 v13.59,49.29
GPIO27
  Top 0.305: JP1.2 76.48,29.71 77.22,28.97 77.22,12.54 R2.2
H1  (via drill 0.89 pad 1.27)  (3 unrouted)
  other vias: 44.32,36.97 46.86,36.97 41.78,36.97 39.24,36.97
IO2  (via drill 0.33)
  Top 0.254: 328P.32 21.96,28.2 v22.22,28.46 | SV2.2 46.86,40.28 46.1,39.51 37.72,39.51 37.08,40.15 33.15,40.15 31.62,41.67 24.13,41.67 20.32,37.86 20.32,36.59 v19.75,36.02
  Bottom 0.254: v22.22,28.46 22.22,28.72 21.84,29.1 21.84,33.93 20.13,35.64 v19.75,36.02 19.3,36.47 17.23,36.47 U$3.2
IO3  (via drill 0.33)
  Top 0.254: SV2.3 47.24,39.01 37.72,39.01 36.83,38.12 34.42,38.12 31.37,41.16 24.38,41.16 20.83,37.61 20.83,33.54 v19.68,32.4 | v19.94,28.59 19.94,28.21 19.56,27.83 19.56,26.21 328P.1
  Bottom 0.254: v19.68,32.4 19.68,28.85 v19.94,28.59
IO4
  Top 0.254: 328P.2 19.72,24.5 19.05,25.16 19.05,30.5 20.57,32.02 20.57,32.27 21.34,33.04 21.34,37.35 24.64,40.66 31.11,40.66 34.16,37.61 34.16,36.85 34.93,36.08 36.45,36.08 37.08,36.72 37.08,37.61 37.97,38.5 49.28,38.5 SV2.4
IO5/COLD_RESET  (via drill 0.33)
  Top 0.254: 328P.9 20.04,16.27 12.7,16.27 7.11,21.86 S1.1 7.35,25.4 7.35,25.42 15.49,25.42 17.53,27.45 17.53,29.86 18.8,31.13 18.8,37.1 23.88,42.18 v37.72,42.18
  Bottom 0.254: SV2.6 57.02,41.93 56.26,42.69 38.23,42.69 v37.72,42.18
IO6/BEE_RXD  (via drill 0.33)
  Top 0.254: U6.6 30.6,13.47 v31.37,14.24 | v31.37,14.24 32,13.61 32.89,13.61 33.27,13.61 v33.4,13.73 | v37.72,13.61 38.48,12.84 42.93,12.84 43.56,13.48 45.09,13.48 SV1.2 | BEE1.3 13.96,43.07 19.94,43.07 20.7,42.31 v21.46,42.31 | 328P.10 22.77,16.88 23.49,16.15 29.46,16.15 v31.37,14.24
  Bottom 0.254: v33.4,13.73 33.53,13.61 v37.72,13.61 | v31.37,14.24 31.37,28.59 27.81,32.15 27.81,33.93 22.61,39.13 22.61,41.16 v21.46,42.31
IO7/BEE_TXD  (via drill 0.33)
  Top 0.254: U6.5 32.11,12.74 v32.13,12.72 | BEE1.2 14.32,45.13 15.75,43.7 v21.72,43.7 | 328P.11 23.56,17.22 24.13,16.65 29.34,16.65 29.84,17.16 32,17.16 32.51,16.65 v32.64,16.78
  Bottom 0.254: 31.88,16.65 31.88,28.85 28.32,32.4 28.32,34.18 23.11,39.39 23.11,42.31 v21.72,43.7 | 31.88,16.65 31.88,15.26 32.51,14.62 32.51,13.61 32.13,13.22 v32.13,12.72 32.26,12.84 34.04,12.84 34.16,12.72 42.8,12.72 43.56,13.48 47.62,13.48 SV1.3 | v32.64,16.78 32,16.78 31.88,16.65
IO9  (via drill 0.33)
  Top 0.254: 328P.13 25.16,19.05 v24.64,19.57 | v22.48,36.34 22.48,37.74 24.89,40.15 30.86,40.15 33.66,37.35 33.66,35.7 35.18,34.18 36.83,34.18 38.35,35.7 57.66,35.7 58.29,36.34 58.29,37.99 59.69,39.39 59.69,41.04 SV2.7
  Bottom 0.254: v24.64,19.57 24.51,19.7 24.51,24.4 24.77,24.65 24.77,32.02 24.26,32.53 24.26,34.56 v22.48,36.34
LED_CTL
  Top 0.254: 328P.12 24.36,17.43 24.64,17.16 29.08,17.16 29.59,17.67 33.98,17.67 R31.1
MISO  (via drill 0.33)
  Top 0.254: v28.45,18.05 27.94,18.05 27.79,18.2 328P.16 27.69,18.32 27.69,19.7 26.29,21.1 22.61,21.1 v21.84,20.34 | ICSP.1 16.26,9.41 18.03,7.64 20.7,7.64 21.34,7 21.34,4.85 ROUTER.7
  Bottom 0.254: v28.45,18.05 27.3,16.91 27.3,11.7 23.88,8.27 23.88,4.59 22.86,3.57 ROUTER.7 | v21.84,20.34 21.34,20.84 21.34,32.4 19.18,34.56 17.22,34.56 U$3.1
MOSI  (via drill 0.33)
  Top 0.254: 26.8,18.17 328P.15 26.8,18.23 v26.8,19.45 | v27.3,38.12 27.3,37.86 v24.89,35.45
  Bottom 0.254: ROUTER.8 22.61,6.88 23.37,7.64 23.37,8.53 24.77,9.92 24.77,10.3 24.39,10.68 24.39,11.58 25.4,12.59 25.4,13.35 24.89,13.86 24.89,14.11 | 24.89,14.11 24.89,14.24 25.65,15 26.29,15 26.8,15.51 v26.8,19.45 26.67,19.57 26.67,21.23 26.16,21.73 26.16,23.38 26.42,23.64 26.42,24.4 26.16,24.65 26.16,31.51 26.67,32.02 26.67,33.04 25.91,33.8 25.4,33.8 24.89,34.31 v24.89,35.45 | ICSP.4 14.99,13.35 17.14,13.35 17.91,14.11 24.89,14.11 | U$3.12 27.7,38.51 v27.3,38.12
MS14_RESET
  Top 0.254: ROUTER.3 17.53,3.69 16.26,4.97 16.26,7.13 14.99,8.4 14.99,12.72 14.35,13.35 13.08,13.35 11.3,15.13 9.52,15.13 S1.4
N$2  (via drill 0.89 pad 1.27)  (1 unrouted)
  other vias: 49.4,36.97 51.94,36.97
N$3  (via drill 0.89 pad 1.27)  (1 unrouted)
  other vias: 54.48,36.97 57.02,36.97
N$4
  Top 0.254: T1.2 22.21,11.84 22.73,11.32 22.73,9.36 R1.2 R4.2
N$5  (via drill 0.89 pad 1.27)  (1 unrouted)
  other vias: 59.56,36.97 62.1,36.97
N$7  (via drill 0.89 pad 1.27)  (1 unrouted)
  other vias: 64.64,36.97 67.18,36.97
N$8
  Top 0.254: T2.2 19.04,10.09 R15.2 R5.1
N$9
  Top 0.254: R31.2 R30.2 T3.2
N$10  (via drill 0.89 pad 1.27)  (2 unrouted)
  other vias: 69.72,36.97 72.26,36.97 74.8,36.97
N$11
  Top 0.203: R2.1 R7.2 73.99,11.12 T4.2
N$12
  Top 0.305: T5.2 8.04,33.91 R11.1 R12.2
N$13  (via drill 0.89 pad 1.27)  (3 unrouted)
  other vias: 44.32,34.43 46.86,34.43 41.78,34.43 39.24,34.43
N$14  (via drill 0.89 pad 1.27)  (1 unrouted)
  other vias: 49.4,34.43 51.94,34.43
N$15  (via drill 0.89 pad 1.27)  (1 unrouted)
  other vias: 54.48,34.43 57.02,34.43
N$16  (via drill 1.02)
  Top 0.61: 35.7,50.95 I-PEX.SIG 34.39,49.42 v34.04,49.42
  Bottom 0.254: 32.89,46.5 33.16,46.5 U$3.8 33.77,46.51 33.78,46.5 34.04,46.5
  Bottom 0.61: 34.04,46.5 v34.04,49.42
N$17  (via drill 0.89 pad 1.27)  (1 unrouted)
  other vias: 59.56,34.43 62.1,34.43
N$18  (via drill 0.89 pad 1.27)  (1 unrouted)
  other vias: 64.64,34.43 67.18,34.43
N$19  (via drill 0.89 pad 1.27)  (2 unrouted)
  other vias: 69.72,34.43 72.26,34.43 74.8,34.43
N$20  (via drill 0.89 pad 1.27)  (3 unrouted)
  other vias: 44.32,31.89 46.86,31.89 41.78,31.89 39.24,31.89
N$21  (via drill 0.89 pad 1.27)  (1 unrouted)
  other vias: 49.4,31.89 51.94,31.89
N$22  (via drill 0.89 pad 1.27)  (1 unrouted)
  other vias: 54.48,31.89 57.02,31.89
N$23  (via drill 0.89 pad 1.27)  (1 unrouted)
  other vias: 59.56,31.89 62.1,31.89
N$24  (via drill 0.89 pad 1.27)
  other vias: 64.64,31.89
N$25  (via drill 0.89 pad 1.27)  (3 unrouted)
  other vias: 44.32,29.35 46.86,29.35 41.78,29.35 39.24,29.35
N$26  (via drill 0.89 pad 1.27)  (1 unrouted)
  other vias: 49.4,29.35 51.94,29.35
N$27  (via drill 0.89 pad 1.27)  (1 unrouted)
  other vias: 54.48,29.35 57.02,29.35
N$28  (via drill 0.89 pad 1.27)  (1 unrouted)
  other vias: 59.56,29.35 62.1,29.35
N$29  (via drill 0.89 pad 1.27)
  other vias: 64.64,29.35
N$30  (via drill 0.89 pad 1.27)  (3 unrouted)
  other vias: 44.32,26.81 46.86,26.81 41.78,26.81 39.24,26.81
N$31  (via drill 0.89 pad 1.27)  (1 unrouted)
  other vias: 49.4,26.81 51.94,26.81
N$32  (via drill 0.89 pad 1.27)  (1 unrouted)
  other vias: 54.48,26.81 57.02,26.81
N$33  (via drill 0.89 pad 1.27)  (1 unrouted)
  other vias: 59.56,26.81 62.1,26.81
N$34  (via drill 0.89 pad 1.27)  (1 unrouted)
  other vias: 64.64,26.81 67.18,26.81
N$35  (via drill 0.89 pad 1.27)  (2 unrouted)
  other vias: 69.72,26.81 72.26,26.81 74.8,26.81
N$36  (via drill 0.89 pad 1.27)  (4 unrouted)
  other vias: 46.86,24.27 49.4,24.27 44.32,24.27 41.78,24.27 39.24,24.27
N$37  (via drill 0.89 pad 1.27)  (1 unrouted)
  other vias: 51.94,24.27 54.48,24.27
N$38  (via drill 0.89 pad 1.27)  (1 unrouted)
  other vias: 57.02,24.27 59.56,24.27
N$39  (via drill 0.89 pad 1.27)  (1 unrouted)
  other vias: 62.1,24.27 64.64,24.27
N$40  (via drill 0.89 pad 1.27)  (3 unrouted)
  other vias: 67.18,24.27 69.72,24.27 72.26,24.27 74.8,24.27
N$41  (via drill 0.89 pad 1.27)  (4 unrouted)
  other vias: 46.86,21.73 49.4,21.73 44.32,21.73 41.78,21.73 39.24,21.73
N$42  (via drill 0.89 pad 1.27)  (1 unrouted)
  other vias: 51.94,21.73 54.48,21.73
N$43  (via drill 0.89 pad 1.27)  (1 unrouted)
  other vias: 57.02,21.73 59.56,21.73
N$44  (via drill 0.89 pad 1.27)  (1 unrouted)
  other vias: 62.1,21.73 64.64,21.73
N$45  (via drill 0.89 pad 1.27)  (3 unrouted)
  other vias: 67.18,21.73 69.72,21.73 72.26,21.73 74.8,21.73
N$46  (via drill 0.89 pad 1.27)  (3 unrouted)
  other vias: 44.32,19.19 46.86,19.19 41.78,19.19 39.24,19.19
N$47  (via drill 0.89 pad 1.27)  (1 unrouted)
  other vias: 49.4,19.19 51.94,19.19
N$48  (via drill 0.89 pad 1.27)  (1 unrouted)
  other vias: 54.48,19.19 57.02,19.19
N$49  (via drill 0.89 pad 1.27)  (1 unrouted)
  other vias: 59.56,19.19 62.1,19.19
N$50  (via drill 0.89 pad 1.27)  (1 unrouted)
  other vias: 64.64,19.19 67.18,19.19
N$51  (via drill 0.89 pad 1.27)  (2 unrouted)
  other vias: 69.72,19.19 72.26,19.19 74.8,19.19
N$52  (via drill 0.89 pad 1.27)  (3 unrouted)
  other vias: 44.32,16.65 46.86,16.65 41.78,16.65 39.24,16.65
N$53  (via drill 0.89 pad 1.27)  (1 unrouted)
  other vias: 49.4,16.65 51.94,16.65
N$54  (via drill 0.89 pad 1.27)  (1 unrouted)
  other vias: 54.48,16.65 57.02,16.65
N$55  (via drill 0.89 pad 1.27)  (1 unrouted)
  other vias: 59.56,16.65 62.1,16.65
N$56  (via drill 0.89 pad 1.27)  (1 unrouted)
  other vias: 64.64,16.65 67.18,16.65
N$57  (via drill 0.89 pad 1.27)  (2 unrouted)
  other vias: 69.72,16.65 72.26,16.65 74.8,16.65
SCK  (via drill 0.33)
  Top 0.254: 328P.17 29.21,19.54 29.59,19.54 v29.59,18.56 | v28.7,36.85 27.94,36.85 v25.78,34.69 | ICSP.3 17.02,12.08 17.65,11.45 17.65,8.91 18.41,8.14 20.95,8.14 21.59,7.51 23.76,7.51 ROUTER.10
  Bottom 0.254: ROUTER.10 25.02,6.25 25.02,8.53 27.81,11.32 27.81,16.65 28.32,17.16 28.83,17.16 29.59,17.92 v29.59,18.56 29.08,19.07 29.08,20.59 28.19,21.48 27.3,21.48 26.67,22.11 26.67,23.13 26.92,23.38 26.92,24.65 26.67,24.91 26.67,31.26 27.18,31.77 27.18,33.29 v25.78,34.69 | U$3.13 33,36.34 33.02,36.34 32.51,36.85 v28.7,36.85
SENSOR_LED  (via drill 0.33)
  Top 0.254: ROUTER.16 32.89,6.23 32.89,8.4 33.4,8.91 v33.4,10.18 | v33.4,11.95 34.12,12.67 34.12,13.03 T3.1
  Bottom 0.254: v33.4,11.95 v33.4,10.18
SS  (via drill 0.33)
  Top 0.254: 328P.14 25.96,19.9 v25.65,20.21 | S1.2 4.57,27.19 v5.59,28.21 | v20.45,26.81 21.59,25.67 21.59,24.91 21.97,24.53 23.11,24.53 23.49,24.15 25.15,24.15 v25.4,23.89 | v29.72,35.96 28.7,35.96 v25.53,32.78
  Bottom 0.254: v25.65,20.21 25.65,24.15 25.65,32.66 v25.53,32.78 | 33,34.69 U$3.14 33.13,34.56 31.37,34.56 29.97,35.96 v29.72,35.96 | v20.45,26.81 10.92,26.81 9.52,28.21 v5.59,28.21
  Bottom 0.305: v25.4,23.89 25.65,24.15
UART_RXD
  Top 0.254: ROUTER.14 30.1,6.11 28.57,7.64 27.56,7.64 26.54,8.65 U2.2
  Top 0.305: U6.2 30.1,6.11 ROUTER.14
UART_RXD1  (via drill 0.33)
  Top 0.254: U2.6 27.05,14.37 26.29,15.13 22.1,15.13 v21.97,15 | v23.88,25.04 23.62,25.29 23.62,26.73 328P.30
  Bottom 0.254: v21.97,15 21.97,16.15 22.61,16.78 22.61,18.3 23.75,19.45 23.75,24.91 v23.88,25.04
UART_TXD
  Top 0.305: ROUTER.13 30.61,3.57 31.5,4.46 31.5,7.13 30.61,8.02 U6.3 30.6,10.68 27.05,10.68 U2.3
  Bottom 0.203: 30.23,3.57 ROUTER.13
UART_TXD1  (via drill 0.33)
  Top 0.254: U2.5 27.55,14.63 26.54,15.64 22.73,15.64 22.48,15.89 21.46,15.89 v20.83,15.26 | v22.73,25.42 22.73,26.76 328P.31
  Bottom 0.254: v22.73,25.42 22.35,25.04 22.35,21.73 23.24,20.84 23.24,19.7 22.1,18.56 22.1,17.03 20.83,15.76 v20.83,15.26
XTAL1
  Top 0.254: 328P.7 20.44,20.53 R16.2 17.36,21.1 15.24,21.1 15.26,21.08 Y1.3
XTAL2
  Top 0.203: 328P.8 20.39,19.62
  Top 0.254: 20.39,19.62 R16.1 17.4,19.08 Y1.1

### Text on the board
tDocu: 7A | 1A | 7B | 1B | BEE SOCKET | GND | 2 | #3 | 4 | GND | #5 | #9 | AREF | Model: M328W V1.0 | DIGITAL [#PWM] | SS | SS<-->MS14 | MS14_RST<-->IO5 | DIGITAL IO | ANALOG IN | GND | ~ | RST | 3V3 | #6 | 7 | GND | A0 | A1 | A2 | A3 | A4 | A5 | MOSI | SCK | 3V3 | MISO | 5V | Wireless IoT Module
214bmp: D:/SmartProjects/Snc/a4_bn_logo2.bmp

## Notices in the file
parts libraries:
frames: http://creativecommons.org/licenses/by-sa/3.0
frames: Released under the CC Attribution Share-Alike 3.0 License
